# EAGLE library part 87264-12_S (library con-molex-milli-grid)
RECEPTACAL
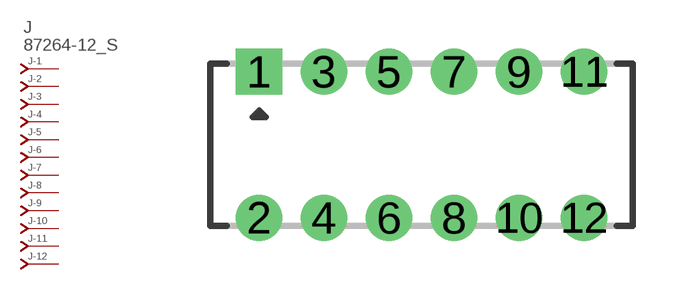
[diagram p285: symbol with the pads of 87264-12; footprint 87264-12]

Designator prefix J; gates -1=J-NV -2=J-N -3=J-N -4=J-N -5=J-N -6=J-N -7=J-N -8=J-N -9=J-N -10=J-N -11=J-N -12=J-N

## 87264-12_S  [87264-12]
1  -1:J  pas
2  -2:J  pas
3  -3:J  pas
4  -4:J  pas
5  -5:J  pas
6  -6:J  pas
7  -7:J  pas
8  -8:J  pas
9  -9:J  pas
10  -10:J  pas
11  -11:J  pas
12  -12:J  pas

## Footprint 87264-12 (pad centres in mm)
RECEPTACAL Dual Row, Side Entry
drill 0.914 square: 1 -5,2.25
drill 0.914: 2 -5,-2.25; 3 -3,2.25; 4 -3,-2.25; 5 -1,2.25; 6 -1,-2.25; 7 1,2.25; 8 1,-2.25; 9 3,2.25; 10 3,-2.25; 11 5,2.25; 12 5,-2.25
